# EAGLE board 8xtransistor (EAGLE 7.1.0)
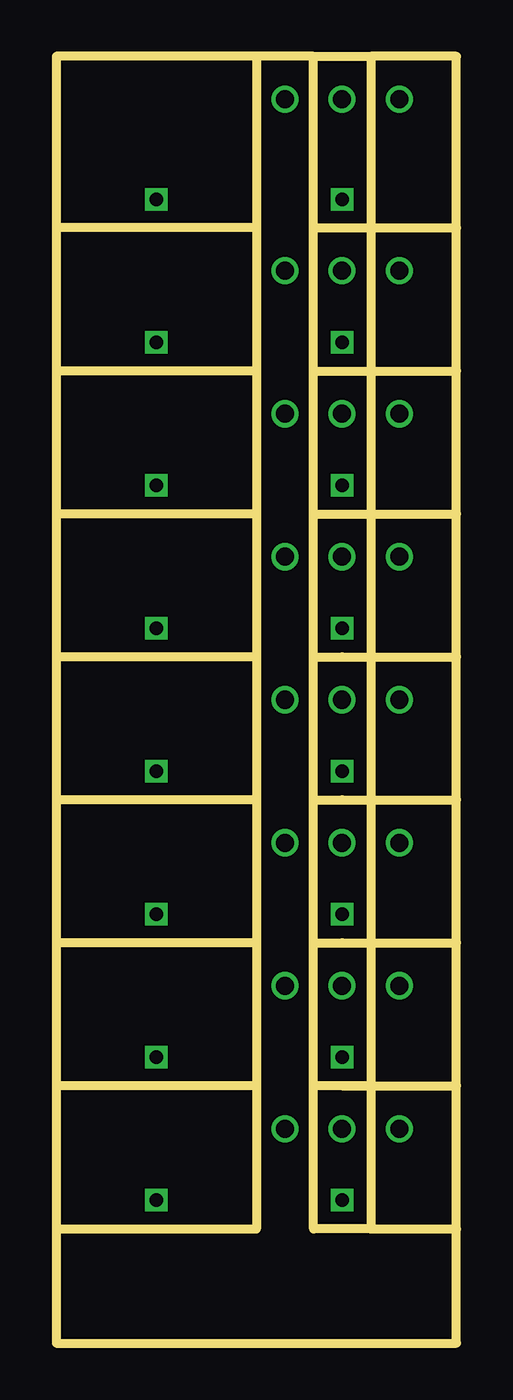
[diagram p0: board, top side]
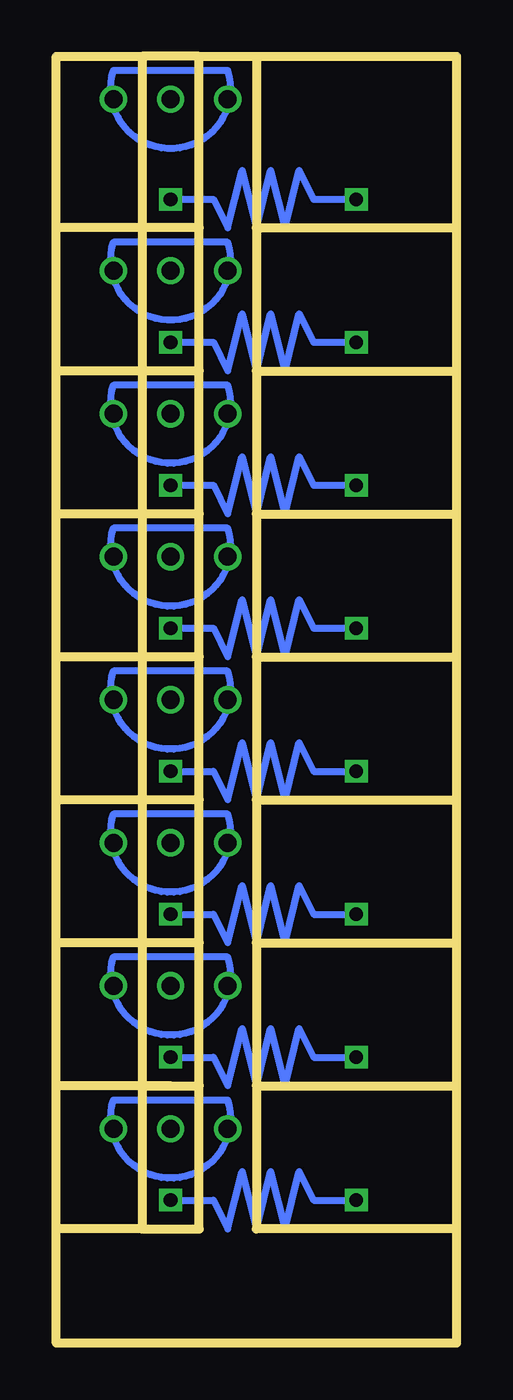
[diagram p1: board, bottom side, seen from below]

Size 17.78 x 57.15 mm. Coordinates in mm from the lower left corner, seen from the top.
Outline: 83 segments
Copper layers (1*16): Top 0.035mm / dielectric 1.5mm / Bottom 0.035mm
Design rules "default": minimum track width 10mil, minimum drill 24mil, track to track 8mil, track to pad 8mil, pad to pad 8mil, via to via 8mil, smd to smd 8mil, copper to edge 40mil, drill to drill 8mil, minimum pad ring 10mil, minimum via ring 8mil, stop-mask expansion 4mil, vias tented up to drill 0mil, thermal gap 10mil

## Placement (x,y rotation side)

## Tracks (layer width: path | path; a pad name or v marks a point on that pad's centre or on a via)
S$1
  Bottom 0.305: 10.16,36.2 15.24,36.2 arc-215 10.16,36.2
S$2  (via drill 0.8)
  other vias: 12.7,34.92 15.24,34.92 10.16,34.92
S$3
  Bottom 0.305: 10.16,10.79 15.24,10.79 arc-215 10.16,10.79
S$4  (via drill 0.8)
  other vias: 12.7,9.53 15.24,9.53 10.16,9.53
S$5
  Bottom 0.305: 10.16,17.14 15.24,17.14 arc-215 10.16,17.14
S$6  (via drill 0.8)
  other vias: 12.7,15.88 15.24,15.88 10.16,15.88
S$7
  Bottom 0.305: 10.16,23.5 15.24,23.5 arc-215 10.16,23.5
S$8  (via drill 0.8)
  other vias: 12.7,22.23 15.24,22.23 10.16,22.23
S$9
  Bottom 0.305: 10.16,29.84 15.24,29.84 arc-215 10.16,29.84
S$10  (via drill 0.8)
  other vias: 12.7,28.57 15.24,28.57 10.16,28.57
S$11
  Bottom 0.305: 10.16,42.55 15.24,42.55 arc-215 10.16,42.55
S$12  (via drill 0.8)
  other vias: 12.7,41.27 15.24,41.27 10.16,41.27
S$13
  Bottom 0.305: 10.16,48.9 15.24,48.9 arc-215 10.16,48.9
S$14  (via drill 0.8)
  other vias: 12.7,47.62 15.24,47.62 10.16,47.62
S$15
  Bottom 0.305: 10.16,56.52 15.24,56.52 arc-215 10.16,56.52
S$16  (via drill 0.8)
  other vias: 12.7,55.24 15.24,55.24 10.16,55.24
S$17  (via drill 0.6)
  Bottom 0.305: v12.7,6.35 10.79,6.35 10.16,5.08 9.53,7.62 8.89,5.08 8.26,7.62 7.62,5.08 6.99,7.62 6.35,6.35 v4.45,6.35
S$18  (via drill 0.6)
  Bottom 0.305: v12.7,12.7 10.79,12.7 10.16,11.43 9.53,13.97 8.89,11.43 8.26,13.97 7.62,11.43 6.99,13.97 6.35,12.7 v4.45,12.7
S$20  (via drill 0.6)
  Bottom 0.305: v12.7,19.05 10.79,19.05 10.16,17.78 9.53,20.32 8.89,17.78 8.26,20.32 7.62,17.78 6.99,20.32 6.35,19.05 v4.45,19.05
S$21  (via drill 0.6)
  Bottom 0.305: v12.7,31.75 10.79,31.75 10.16,30.48 9.53,33.02 8.89,30.48 8.26,33.02 7.62,30.48 6.99,33.02 6.35,31.75 v4.45,31.75
S$22  (via drill 0.6)
  Bottom 0.305: v12.7,38.1 10.79,38.1 10.16,36.83 9.53,39.37 8.89,36.83 8.26,39.37 7.62,36.83 6.99,39.37 6.35,38.1 v4.45,38.1
S$23  (via drill 0.6)
  Bottom 0.305: v12.7,44.45 10.79,44.45 10.16,43.18 9.53,45.72 8.89,43.18 8.26,45.72 7.62,43.18 6.99,45.72 6.35,44.45 v4.45,44.45
S$24  (via drill 0.6)
  Bottom 0.305: v12.7,50.8 10.79,50.8 10.16,49.53 9.53,52.07 8.89,49.53 8.26,52.07 7.62,49.53 6.99,52.07 6.35,50.8 v4.45,50.8
S$25  (via drill 0.6)
  Bottom 0.305: v12.7,25.4 10.79,25.4 10.16,24.13 9.53,26.67 8.89,24.13 8.26,26.67 7.62,24.13 6.99,26.67 6.35,25.4 v4.45,25.4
